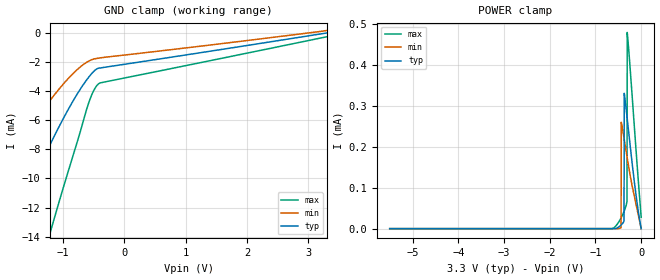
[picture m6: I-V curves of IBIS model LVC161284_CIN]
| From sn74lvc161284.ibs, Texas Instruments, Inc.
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[Model]   LVC161284_CIN
Model_type  Input
Vinl=0.8
Vinh=2.3
| variable   typ   min   max
C_comp   1.18pF   0.92pF   1.48pF
[Temperature Range]   40   100   -40
| Ambient temperature   25   85   -40
[Voltage range]   3.3   3   3.6
[GND Clamp]
| LVC161284_CIN
|   Voltage   I(typ)   I(min)   I(max)
-5.5V     -53.56mA   -34.69mA   -89.34mA
-2.58V    -21.28mA   -13.57mA   -36.36mA
-1.845V   -13.71mA   -8.554mA   -23.87mA
-1.775V   -13.02mA   -8.099mA   -22.72mA
-1.46V    -9.993mA   -6.124mA   -17.67mA
-1.23V    -7.91mA    -4.783mA   -14.15mA
-1.175V   -7.432mA   -4.479mA   -13.33mA
-840mV    -4.752mA   -2.834mA   -8.571mA
-575mV    -3.043mA   -1.937mA   -4.808mA
-490mV    -2.63mA    -1.79mA    -3.936mA
-405mV    -2.417mA   -1.726mA   -3.471mA
3.3V      142.9pA    168.7uA    -261.4uA
[POWER Clamp]
| LVC161284_CIN
|   Voltage   I(typ)   I(min)   I(max)
-5.5V     9.359nA    26.89nA    1.244nA
-585mV    12.05nA    601.7pA    3.285uA
-440mV    8.724uA    2.43uA     26.26uA
-435mV    9.268uA    259.4uA    27.35uA
-375mV    19.07uA    220.6uA    42.01uA
-370mV    330uA      217.2uA    43.39uA
-310mV    273uA      175.5uA    67.35uA
-305mV    267.9uA    172.1uA    478.3uA
-250mV    212.1uA    135.7uA    403.5uA
-130mV    96.77uA    68.64uA    218.4uA
-70mV     47.77uA    36.99uA    127.7uA
-95.1fV   142.9pA    581.3pA    27.84uA
